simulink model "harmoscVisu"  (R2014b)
settings: Solver=ode45  StartTime=0.0  StopTime=10.0  RelTol=1e-3
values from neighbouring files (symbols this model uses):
  omega = 2*pi/(24*3600)    (= 7.27220521664e-05)    [foucault_call.m]    (also in GravWirk.m = 1)

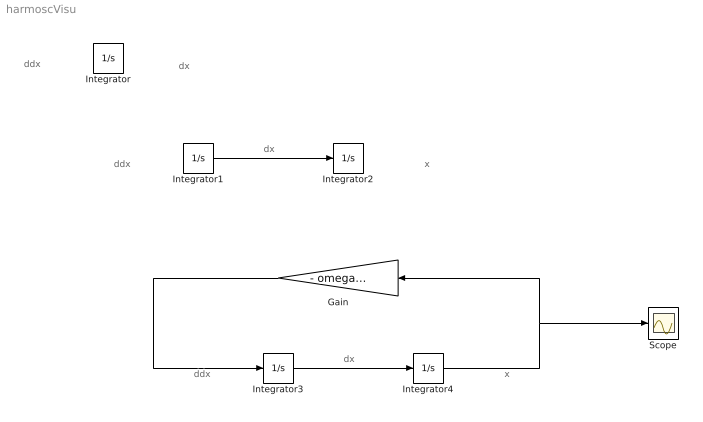
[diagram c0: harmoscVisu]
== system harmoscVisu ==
  note: x
  note: dx
  note: ddx
  note: dx
  note: ddx
  note: x
  note: dx
  note: ddx
  Gain : Gain  Gain=- omega.^2
  Integrator{,1..2,4} (4 alike) : Integrator
  Integrator3 : Integrator  InitialCondition=1
  Scope : Scope
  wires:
  Integrator/1 -> ?
  ? -> Integrator/1
  Integrator1/1 -> Integrator2/1
  ? -> Integrator1/1
  Integrator2/1 -> ?
  Integrator3/1 -> Integrator4/1
  Integrator4/1 -> Scope/1, Gain/1
  Gain/1 -> Integrator3/1
